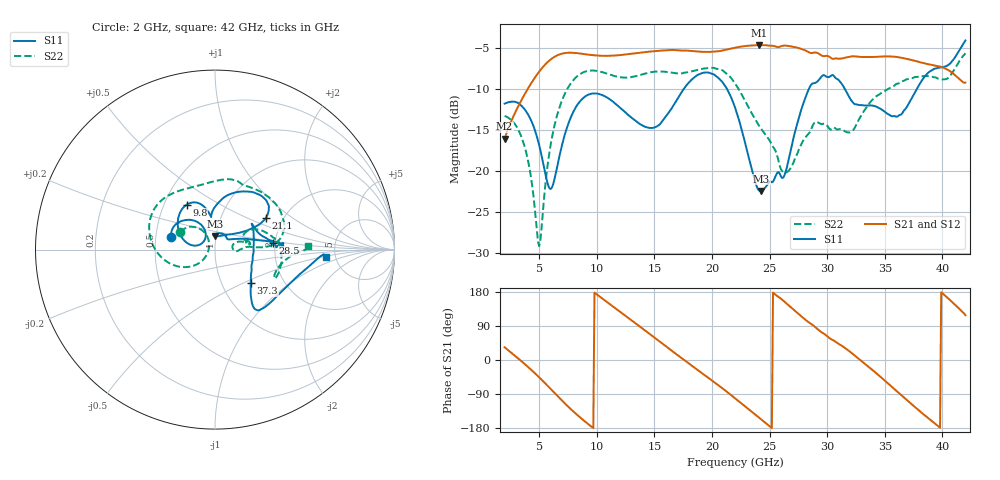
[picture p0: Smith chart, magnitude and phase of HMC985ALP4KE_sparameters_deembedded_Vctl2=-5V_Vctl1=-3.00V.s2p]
!s2p File: Measurements: S11, S21, S12, S22
# GHz S dB R 50.0
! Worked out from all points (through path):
!   401 points, 2 GHz to 42 GHz, reference 50 ohm
!   highest |S21| = -4.70 dB at 24.1 GHz (marker M1); lowest = -16.1 dB at 2 GHz (marker M2)
!   lowest |S11| = -22.4 dB at 24.3 GHz (marker M3), VSWR 1.16, Z = 49.6 + j7.54 ohm
!   |S11| at or under -10 dB: start of sweep to 17.57 GHz; 21.29 GHz to 28.43 GHz (7.135 GHz wide, 28.7 % of centre); 31.52 GHz to 37.8 GHz (6.283 GHz wide, 18.1 % of centre)
!   |S22| runs from -29.2 to -5.7 dB; largest |S21 - S12| = 0.00067
!   S11 on the Smith chart (normalised r, x): 2 GHz: 0.60, +0.09; 9.8 GHz: 0.65, +0.36; 21.1 GHz: 1.63, +0.64; 28.5 GHz: 1.94, +0.16; 37.3 GHz: 1.37, -0.55; 42 GHz: 4.20, -0.56
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2  -11.82 163.5  -16.09 33.6  -16.09 33.6  -13.31 153.2
3.7  -12.45 137.0  -10.78 -9.4  -10.79 -9.4  -16.88 126.2
5  -16.87 117.9  -7.93 -45.7  -7.93 -45.7  -29.16 170.7
6.1  -22.04 150.6  -6.34 -79.7  -6.34 -79.7  -16.02 -144.2
7.2  -15.71 166.1  -5.68 -113.7  -5.68 -113.7  -10.71 -169.4
8.7  -11.31 138.5  -5.76 -155.3  -5.76 -155.3  -8.11 158.4
9.8  -10.58 122.0  -5.95 177.9  -5.96 177.9  -7.81 140.6
12.9  -13.39 100.1  -5.78 107.5  -5.78 107.5  -8.62 99.6
15.4  -14.43 96.3  -5.40 50.2  -5.40 50.2  -7.92 74.5
18  -9.25 68.6  -5.39 -9.3  -5.39 -9.3  -7.97 59.8
21.1  -9.59 31.7  -5.30 -79.2  -5.30 -79.1  -7.98 16.3
22  -12.28 29.7  -5.02 -100.9  -5.02 -100.9  -9.35 6.3
24.1  -22.41 80.0  -4.70 -152.4  -4.71 -152.3  -14.53 4.7
24.3  -22.43 88.7  -4.70 -157.3  -4.70 -157.3  -14.93 4.8
26.3  -20.50 37.0  -4.77 153.4  -4.77 153.5  -20.21 6.5
28.5  -9.78 6.6  -5.64 97.4  -5.64 97.4  -15.27 15.3
28.7  -9.38 3.5  -5.66 93.4  -5.67 93.4  -14.63 15.1
32.4  -11.88 23.9  -6.07 11.5  -6.07 11.5  -14.74 28.2
35.4  -13.18 9.6  -6.08 -64.9  -6.08 -64.9  -9.96 14.5
37.3  -11.28 -43.1  -6.51 -115.8  -6.51 -115.7  -8.71 -0.9
39.7  -7.45 -49.4  -7.28 -176.3  -7.28 -176.2  -8.79 -25.4
42  -4.14 -3.8  -9.26 118.1  -9.27 118.2  -5.69 2.3
